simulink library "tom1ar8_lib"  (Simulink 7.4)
settings: Solver=ode45  SolverMode=SingleTasking  StartTime=0.0  StopTime=10.0  RelTol=1e-3
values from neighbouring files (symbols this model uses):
  baud = 250000    [MISOcontrol.m]    (also in MISO_demo.m; runSteptest.m; SISOcontrol.m; init.m)
  com = 'COM4'    [MISOcontrol.m]    (also in MISO_demo.m; runSteptest.m; SISOcontrol.m; init.m)
  fTf = 0.1    [MISOcontrol.m]    (also in MISO_demo.m; runSteptest.m; SISOcontrol.m; init.m)
  fTl = 0.05    [MISOcontrol.m]    (also in MISO_demo.m; runSteptest.m; SISOcontrol.m; init.m)
  fTt = 0.05    [MISOcontrol.m]    (also in MISO_demo.m; runSteptest.m; SISOcontrol.m; init.m)
  Ts = 0.1    [identification.m]    (also in MISOcontrol.m; MISO_demo.m; runSteptest.m; SISOcontrol.m)

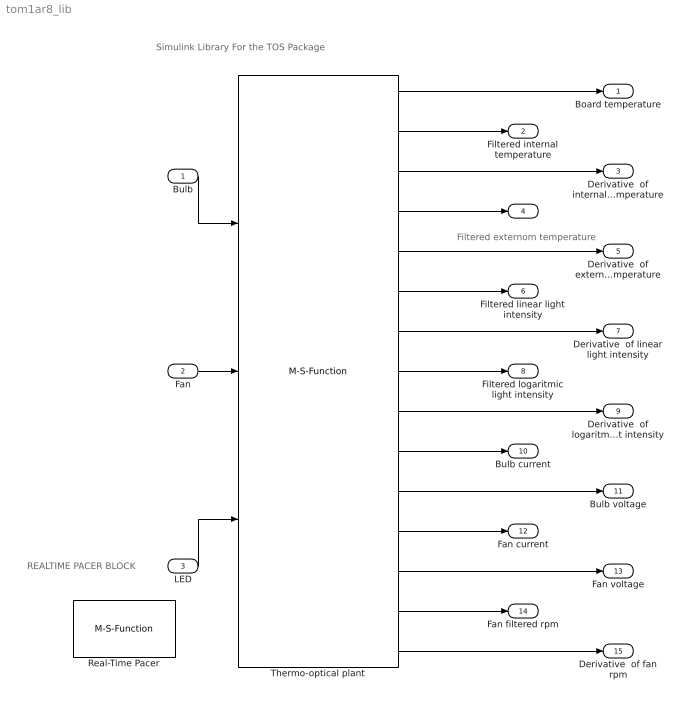
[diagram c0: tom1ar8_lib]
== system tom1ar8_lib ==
  note: Simulink Library For the TOS Package
  note: REALTIME PACER BLOCK
  note: Filtered externom temperature
  Bulb : Inport  OutDataType=fixdt(1, 16)  OutScaling=2^0
  Fan : Inport  Port=2  OutDataType=fixdt(1, 16)  OutScaling=2^0
  LED : Inport  Port=3  OutDataType=fixdt(1, 16)  OutScaling=2^0
  Real-Time Pacer : M-S-Function  FunctionName=msfun_realtime_pacer  Parameters=simTimePerRealTime  mask(RealTime_Pacer){simTimePerRealTime=1}
      mask prompts: simTimePerRealTime "Speedup (Simulation Time / Real Time):"
      mask help: Slow down a simulation to track real (i.e., wall clock) elapsed time. "Speedup" specifies the ratio between simulation time and real time Speedup = N => N sec. of simulation time per sec. of real time Speedup can be fractional (e.g., 0.5, 1.3). Speedup = inf => allow simulation to run at full speed Click on the Help button for details.
  Thermo-optical plant : M-S-Function  FunctionName=tom1ar8  Parameters=Ts,com,baud,fTt,fTl,fTf
  Board temperature : Outport  OutDataType=fixdt(1, 16)  OutScaling=2^0
  Filtered internal temperature : Outport  Port=2  OutDataType=fixdt(1, 16)  OutScaling=2^0
  Derivative  of internal temperature : Outport  Port=3  OutDataType=fixdt(1, 16)  OutScaling=2^0
  " " : Outport  Port=4  OutDataType=fixdt(1, 16)  OutScaling=2^0
  Derivative  of external temperature : Outport  Port=5  OutDataType=fixdt(1, 16)  OutScaling=2^0
  Filtered linear light intensity : Outport  Port=6  OutDataType=fixdt(1, 16)  OutScaling=2^0
  Derivative  of linear light intensity : Outport  Port=7  OutDataType=fixdt(1, 16)  OutScaling=2^0
  Filtered logaritmic light intensity : Outport  Port=8  OutDataType=fixdt(1, 16)  OutScaling=2^0
  Derivative  of logaritmic light intensity : Outport  Port=9  OutDataType=fixdt(1, 16)  OutScaling=2^0
  Bulb current : Outport  Port=10  OutDataType=fixdt(1, 16)  OutScaling=2^0
  Bulb voltage : Outport  Port=11  OutDataType=fixdt(1, 16)  OutScaling=2^0
  Fan current : Outport  Port=12  OutDataType=fixdt(1, 16)  OutScaling=2^0
  Fan voltage : Outport  Port=13  OutDataType=fixdt(1, 16)  OutScaling=2^0
  Fan filtered rpm : Outport  Port=14  OutDataType=fixdt(1, 16)  OutScaling=2^0
  Derivative  of fan rpm : Outport  Port=15  OutDataType=fixdt(1, 16)  OutScaling=2^0
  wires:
  Thermo-optical plant/1 -> Board temperature/1
  Thermo-optical plant/2 -> Filtered internal temperature/1
  Thermo-optical plant/3 -> Derivative  of internal temperature/1
  Thermo-optical plant/4 -> " "/1
  Thermo-optical plant/5 -> Derivative  of external temperature/1
  Thermo-optical plant/6 -> Filtered linear light intensity/1
  Thermo-optical plant/7 -> Derivative  of linear light intensity/1
  Bulb/1 -> Thermo-optical plant/1
  Fan/1 -> Thermo-optical plant/2
  LED/1 -> Thermo-optical plant/3
  Thermo-optical plant/8 -> Filtered logaritmic light intensity/1
  Thermo-optical plant/9 -> Derivative  of logaritmic light intensity/1
  Thermo-optical plant/10 -> Bulb current/1
  Thermo-optical plant/11 -> Bulb voltage/1
  Thermo-optical plant/12 -> Fan current/1
  Thermo-optical plant/13 -> Fan voltage/1
  Thermo-optical plant/14 -> Fan filtered rpm/1
  Thermo-optical plant/15 -> Derivative  of fan rpm/1
